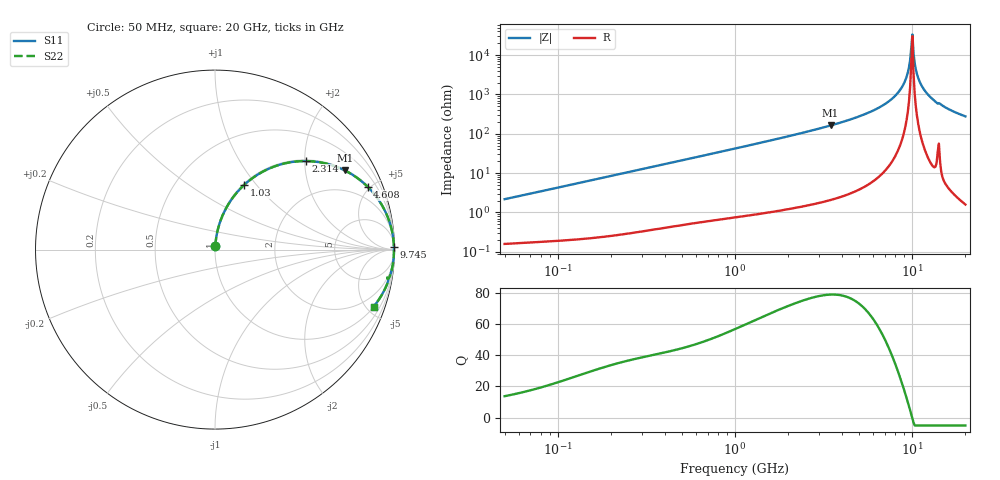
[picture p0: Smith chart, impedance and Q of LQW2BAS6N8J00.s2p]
!Murata Part Number: LQW2BAS6N8J00
!These Parameters are Measured in Series Mode Connection
!  o--[Z]--o
!Port1  Port2
!  o-------o
!Freq. Start=50[MHz] Stop=20[GHz], 401[Steps]
# Hz S RI R 50
!Freq.(Hz) S11(Real) S11(Imag) S21(Real) S21(Imag) S12(Real) S12(Imag) S22(Real) S22(Imag)
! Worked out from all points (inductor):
!   401 points, 50 MHz to 20 GHz, reference 50 ohm
!   read as one part in series: L = 6.86 nH near 51.52 MHz
!   highest Q = 78.7 at 3.467 GHz (marker M1), where L = 7.48 nH
!   self-resonance near 9.892 GHz
!   S11 on the Smith chart (normalised r, x): 50 MHz: 1.00, +0.04; 1.03 GHz: 1.02, +0.87; 2.314 GHz: 1.03, +2.03; 4.608 GHz: 1.06, +4.83; 9.745 GHz: open; 20 GHz: 1.03, -5.54
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5e7  0.00205 0.0216  0.998 -0.0216  0.998 -0.0216  0.00205 0.0216
1.364002e8  0.00545 0.0577  0.9945 -0.0577  0.9945 -0.0577  0.00545 0.0577
3.721004e8  0.0277 0.1524  0.9723 -0.1524  0.9723 -0.1524  0.0277 0.1524
1e9  0.1552 0.3533  0.8448 -0.3533  0.8448 -0.3533  0.1552 0.3533
1.030411e9  0.163 0.3608  0.837 -0.3608  0.837 -0.3608  0.163 0.3608
2.313601e9  0.5064 0.4933  0.4936 -0.4933  0.4936 -0.4933  0.5064 0.4933
2.728004e9  0.597 0.484  0.403 -0.484  0.403 -0.484  0.597 0.484
3.466789e9  0.7238 0.4408  0.2762 -0.4408  0.2762 -0.4408  0.7238 0.4408
4.608136e9  0.8503 0.3502  0.1497 -0.3502  0.1497 -0.3502  0.8503 0.3502
6.034176e9  0.9353 0.2383  0.0647 -0.2383  0.0647 -0.2383  0.9353 0.2383
7.442007e9  0.976 0.1419  0.024 -0.1419  0.024 -0.1419  0.976 0.1419
8.389408e9  0.9897 0.0851  0.0103 -0.0851  0.0103 -0.0851  0.9897 0.0851
9.041845e9  0.9947 0.0492  0.0053 -0.0492  0.0053 -0.0492  0.9947 0.0492
9.457416e9  0.9964 0.0276  0.00355 -0.0276  0.00355 -0.0276  0.9964 0.0276
9.745021e9  0.9971 0.0132  0.00291 -0.0132  0.00291 -0.0132  0.9971 0.0132
9.892087e9  0.9973 0.00596  0.00275 -0.00596  0.00275 -0.00596  0.9973 0.00596
1.019291e10  0.9973 -0.00849  0.00274 0.00849  0.00274 0.00849  0.9973 -0.00849
1.066139e10  0.9965 -0.0302  0.00352 0.0302  0.00352 0.0302  0.9965 -0.0302
1.098561e10  0.9954 -0.0446  0.00457 0.0446  0.00457 0.0446  0.9954 -0.0446
1.238412e10  0.9868 -0.1026  0.0132 0.1026  0.0132 0.1026  0.9868 -0.1026
1.550395e10  0.9534 -0.2053  0.0466 0.2053  0.0466 0.2053  0.9534 -0.2053
2e10  0.8834 -0.3181  0.1166 0.3181  0.1166 0.3181  0.8834 -0.3181
